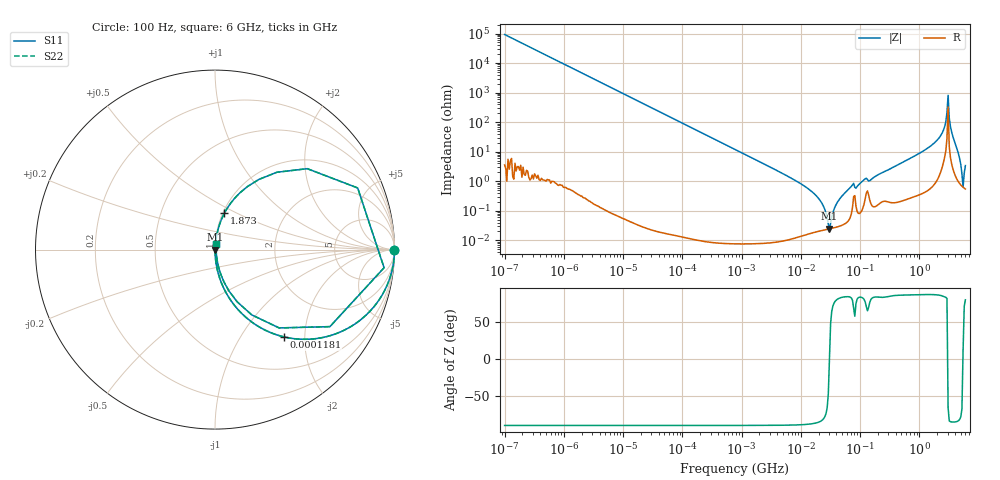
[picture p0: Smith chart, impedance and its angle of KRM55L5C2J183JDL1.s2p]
!Murata Part Number: KRM55L5C2J183JDL1
!These Parameters are Measured in Series Mode Connection
!Data Generated on Jan 08, 2026
!  o--ll--o
!Port1  Port2
!  o------o
!Operation Temp=25[degC], DC Bias Voltage=0[V]
!Freq. Start=100[Hz] Stop=6[GHz] 401[Steps]
# Hz S RI R 50
!Freq.(Hz) S11(Real) S11(Imag) S21(Real) S21(Imag) S12(Real) S12(Imag) S22(Real) S22(Imag)
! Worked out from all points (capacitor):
!   401 points, 100 Hz to 6 GHz, reference 50 ohm
!   read as one part in series: C = 17.1 nF near 109 Hz
!   lowest |Z| = 24.6 mohm at 30.45 MHz (marker M1)
!   series resonance near 30.39 MHz, so ESL is about 1.6 nH
!   S11 on the Smith chart (normalised r, x): 100 Hz: open; 118.1 kHz: 1.00, -1.57; 1.873 GHz: 1.02, +0.43; 6 GHz: 1.01, +0.07
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100  1 -0.00108  1.2e-06 0.00108  1.2e-06 0.00108  1 -0.00108
2008  0.9995 -0.0216  0.000469 0.0216  0.000469 0.0216  0.9995 -0.0216
40335  0.8414 -0.3652  0.1586 0.3652  0.1586 0.3652  0.8414 -0.3652
118133  0.3822 -0.4859  0.6178 0.4859  0.6178 0.4859  0.3822 -0.4859
264476  0.1099 -0.3127  0.8901 0.3127  0.8901 0.3127  0.1099 -0.3127
774597  0.0142 -0.1182  0.9858 0.1182  0.9858 0.1182  0.0142 -0.1182
1.555665e7  0.000197 -0.00436  0.9998 0.00436  0.9998 0.00436  0.000197 -0.00436
2.225763e7  0.000217 -0.00192  0.9998 0.00192  0.9998 0.00192  0.000217 -0.00192
3.045065e7  0.000246 1.16e-05  0.9998 -1.16e-05  0.9998 -1.16e-05  0.000246 1.16e-05
4.165952e7  0.000291 0.00196  0.9997 -0.00196  0.9997 -0.00196  0.000291 0.00196
7.129496e7  0.000829 0.00667  0.9992 -0.00667  0.9992 -0.00667  0.000829 0.00667
3.124326e8  0.00259 0.0254  0.9974 -0.0254  0.9974 -0.0254  0.00259 0.0254
1.873145e9  0.0518 0.202  0.9482 -0.202  0.9482 -0.202  0.0518 0.202
2.34314e9  0.1388 0.3163  0.8612 -0.3163  0.8612 -0.3163  0.1388 0.3163
2.679998e9  0.3448 0.4309  0.6552 -0.4309  0.6552 -0.4309  0.3448 0.4309
2.802721e9  0.5142 0.4508  0.4858 -0.4508  0.4858 -0.4508  0.5142 0.4508
3.065283e9  0.942 -0.101  0.058 0.101  0.058 0.101  0.942 -0.101
3.352442e9  0.3572 -0.4363  0.6428 0.4363  0.6428 0.4363  0.3572 -0.4363
3.8344e9  0.0779 -0.2307  0.9221 0.2307  0.9221 0.2307  0.0779 -0.2307
4.586474e9  0.0162 -0.0816  0.9838 0.0816  0.9838 0.0816  0.0162 -0.0816
5.245841e9  0.00705 -0.0164  0.9929 0.0164  0.9929 0.0164  0.00705 -0.0164
6e9  0.00655 0.0332  0.9934 -0.0332  0.9934 -0.0332  0.00655 0.0332
